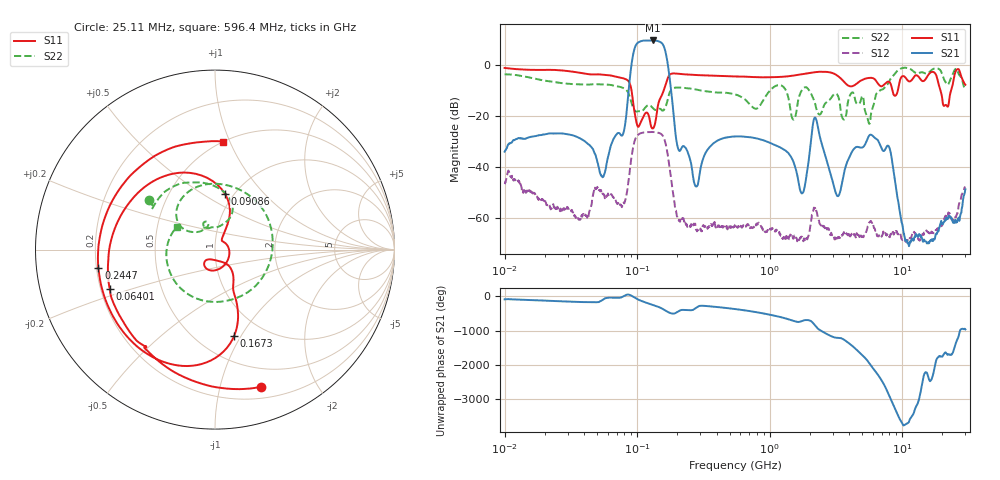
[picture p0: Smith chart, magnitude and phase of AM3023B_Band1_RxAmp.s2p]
# Hz S DB R 50.0
!freq dBS11 angS11 dBS21 angS21 dBS12 angS12 dBS22 angS22
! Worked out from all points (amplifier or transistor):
!   1601 points, 10 MHz to 30 GHz, reference 50 ohm
!   highest |S21| = 9.8 dB at 132.2 MHz (marker M1)
!   |S21| within 3 dB of that: 95.87 MHz to 160.8 MHz (64.92 MHz wide, 50.6 % of centre)
!   unconditionally stable (mu >= 1): start of sweep to end of sweep
!   at 37.85 MHz: K = 5441.20, MAG = -25.0 dB, |S12| = -59.6 dB
!   at 547.7 MHz: K = 9896.16, MAG = -25.6 dB, |S12| = -62.6 dB
!   at 30 GHz: K = 24222.83, MAG = -47.3 dB, |S12| = -47.8 dB
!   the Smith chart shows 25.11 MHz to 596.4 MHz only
!   S11 on the Smith chart (normalised r, x): 25.11 MHz: 0.31, -1.35; 64.01 MHz: 0.24, -0.17; 90.86 MHz: 0.92, +0.63; 167.3 MHz: 0.74, -0.93; 244.7 MHz: 0.21, -0.08; 596.4 MHz: 0.50, +0.95
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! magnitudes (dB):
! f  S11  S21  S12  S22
! 10 MHz  -1.0  -33.9  -46.6  -3.5
! 25.11 MHz  -1.9  -26.7  -55.9  -6.8
! 38.04 MHz  -3.0  -29.0  -59.0  -7.5
! 54.54 MHz  -3.7  -43.8  -49.9  -7.5
! 64.01 MHz  -4.1  -30.9  -50.6  -7.8
! 79.38 MHz  -5.2  -26.0  -53.9  -9.0
! 90.86 MHz  -10.1  0.6  -35.6  -15.0
! 132.2 MHz  -24.7  9.8  -26.2  -16.9
! 144.7 MHz  -15.0  9.5  -26.4  -17.2
! 167.3 MHz  -6.2  2.9  -32.9  -14.9
! 201.3 MHz  -3.3  -31.6  -59.6  -8.7
! 244.7 MHz  -3.6  -35.0  -63.4  -9.0
! 280.1 MHz  -3.8  -47.6  -64.6  -9.5
! 547.7 MHz  -4.4  -27.9  -62.6  -11.4
! 596.4 MHz  -4.4  -27.9  -62.9  -12.1
! 1.758 GHz  -3.5  -50.2  -67.3  -9.6
! 2.084 GHz  -2.9  -26.1  -58.6  -11.9
! 3.269 GHz  -4.2  -51.4  -67.9  -11.9
! 5.584 GHz  -5.0  -27.9  -62.0  -22.5
! 7.926 GHz  -6.4  -31.8  -66.8  -6.6
! 10.97 GHz  -5.8  -69.8  -69.0  -1.1
! 30 GHz  -7.6  -48.6  -47.8  -9.3
